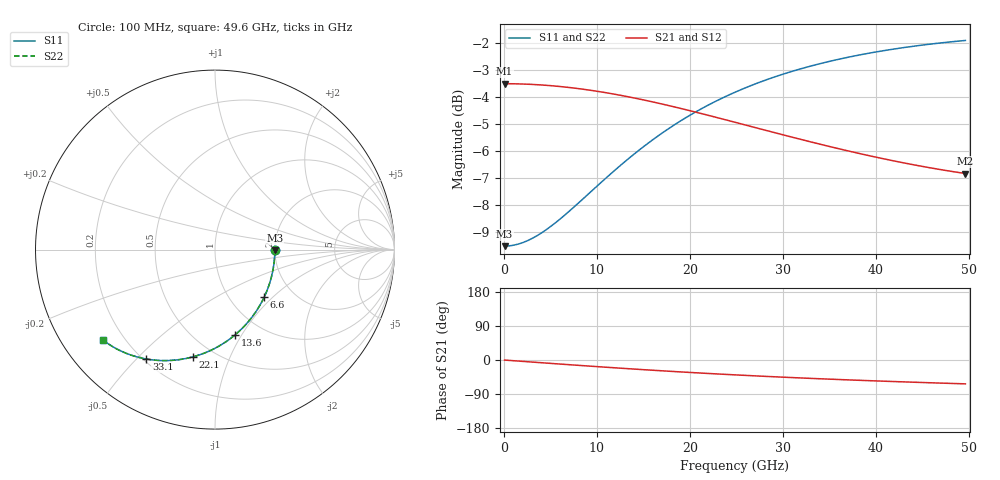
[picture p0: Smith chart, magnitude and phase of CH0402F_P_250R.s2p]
# GHz S RI R 250
! S-Parameters data
! Freq  reS11  imS11  reS21  imS21  reS12  imS12  reS22  imS22
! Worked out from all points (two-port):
!   100 points, 100 MHz to 49.6 GHz, reference 250 ohm
!   highest |S21| = -3.52 dB at 100 MHz (marker M1); lowest = -6.8 dB at 49.6 GHz (marker M2)
!   |S21| within 3 dB of the highest: start of sweep to 43.97 GHz
!   lowest |S11| = -9.5 dB at 100 MHz (marker M3), VSWR 2.00, Z = 500 - j4.74 ohm
!   |S11| at or under -10 dB: nowhere
!   |S22| runs from -9.5 to -1.9 dB; largest |S21 - S12| = 0
!   S11 on the Smith chart (normalised r, x): 100 MHz: 2.00, -0.02; 6.6 GHz: 1.43, -0.89; 13.6 GHz: 0.75, -0.94; 22.1 GHz: 0.39, -0.74; 33.1 GHz: 0.21, -0.53; 49.6 GHz: 0.12, -0.35
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0.1  0.3333 -0.00421  0.6667 -0.00207  0.6667 -0.00207  0.3333 -0.00421
1.6  0.3297 -0.0672  0.6653 -0.0331  0.6653 -0.0331  0.3297 -0.0672
3.1  0.3197 -0.1292  0.6615 -0.0638  0.6615 -0.0638  0.3197 -0.1292
4.6  0.3037 -0.1893  0.6553 -0.0938  0.6553 -0.0938  0.3037 -0.1893
6.6  0.2739 -0.265  0.6437 -0.1326  0.6437 -0.1326  0.2739 -0.265
8.6  0.2354 -0.3344  0.6285 -0.1692  0.6285 -0.1692  0.2354 -0.3344
11.1  0.178 -0.4106  0.6052 -0.2112  0.6052 -0.2112  0.178 -0.4106
12.6  0.1397 -0.4501  0.5893 -0.2343  0.5893 -0.2343  0.1397 -0.4501
13.6  0.1131 -0.4739  0.5781 -0.2487  0.5781 -0.2487  0.1131 -0.4739
15.1  0.072 -0.5057  0.5606 -0.2688  0.5606 -0.2688  0.072 -0.5057
16.6  0.0301 -0.5329  0.5423 -0.2871  0.5423 -0.2871  0.0301 -0.5329
19.1  -0.0403 -0.5687  0.5108 -0.3137  0.5108 -0.3137  -0.0403 -0.5687
20.6  -0.082 -0.5849  0.4917 -0.3273  0.4917 -0.3273  -0.082 -0.5849
22.1  -0.1231 -0.5975  0.4725 -0.3394  0.4725 -0.3394  -0.1231 -0.5975
25.1  -0.2017 -0.6133  0.4349 -0.3592  0.4349 -0.3592  -0.2017 -0.6133
27.1  -0.2511 -0.6177  0.4107 -0.3695  0.4107 -0.3695  -0.2511 -0.6177
29.1  -0.2978 -0.6181  0.3873 -0.3779  0.3873 -0.3779  -0.2978 -0.6181
33.1  -0.3826 -0.6095  0.3435 -0.3898  0.3435 -0.3898  -0.3826 -0.6095
37.1  -0.4561 -0.5915  0.3041 -0.3969  0.3041 -0.3969  -0.4561 -0.5915
41.6  -0.5263 -0.5639  0.2648 -0.4013  0.2648 -0.4013  -0.5263 -0.5639
45.6  -0.5788 -0.5353  0.2341 -0.4034  0.2341 -0.4034  -0.5788 -0.5353
49.6  -0.6232 -0.5043  0.2067 -0.4048  0.2067 -0.4048  -0.6232 -0.5043
